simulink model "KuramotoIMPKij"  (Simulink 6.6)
settings: Solver=ode3  StartTime=0.0  StopTime=Tend  FixedStep=dt  RelTol=1e-8
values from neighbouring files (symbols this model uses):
  A0 = [-1/D1 0 0; 0 0 1; 1 0 0]    [PlatoonDemo.m]    (also in SelfOrgCopterDemo.m = OverallSystd.A; SyncDemo.m = [0 1; 0 0]; SyncIMPDemo.m = [Ai Bi*kri; SyncKuramotoDemo.m = A01)
  B0 = [1/D1; 0; 0]    [PlatoonDemo.m]    (also in SelfOrgCopterDemo.m = OverallSystd.B; SyncDemo.m = [ke1; kr*br1]; SyncIMPDemo.m = [Bi*kei; 1]; SyncKuramotoDemo.m = B01)
  C0 = 0.00001    (= 1e-05)    [LCNetworkDemo.m]    (also in SyncDemo.m; SyncIMPDemo.m = [Ci 0]; SyncKuramotoDemo.m = C01; SyncMotor.m = [C01 zeros(1,n+1); zeros(1,n+1) C02])
  D0 = 0    [SyncDemo.m]    (also in SyncIMPDemo.m; SyncKuramotoDemo.m; SyncMotor.m)
  K = [0:kend-1]    [ConvergenceDemo.m]    (also in DelayDemo.m = inv(diag(-diag(K)))*K; EventtriggeredPendulum.m = lqr(invPendel,q*Q, R, 0); SelfOrgCopterDemo.m = Kneighb; SyncDemo.m = [1 1])
  k = k+1    (= 1)    [charPathLength.m]    (also in SyncKuramotoDemo.m = 0.2)
  n = na+1    (= 3)    [DelayDemo.m]    (also in EventtriggeredPendulum.m = 4; LCLCNetworkDemo.m = 4; LCNetworkDemo.m = 2; PlatoonDemo.m)
  Ni = sum(K')    [SyncKuramotoDemo.m]
  x0 = x0/sum(x0)*N1    [ConsensusDemo.m]    (also in EventtriggeredPendulum.m = [0; 0.18; 0; 0]; LCLCNetworkDemo.m = [x01; zeros((N1-1)*n, 1)]; LCNetworkDemo.m = [1 0 0.5 0 -1 0]; NetwPendulum.m = [0; 0; 0.05; 0])

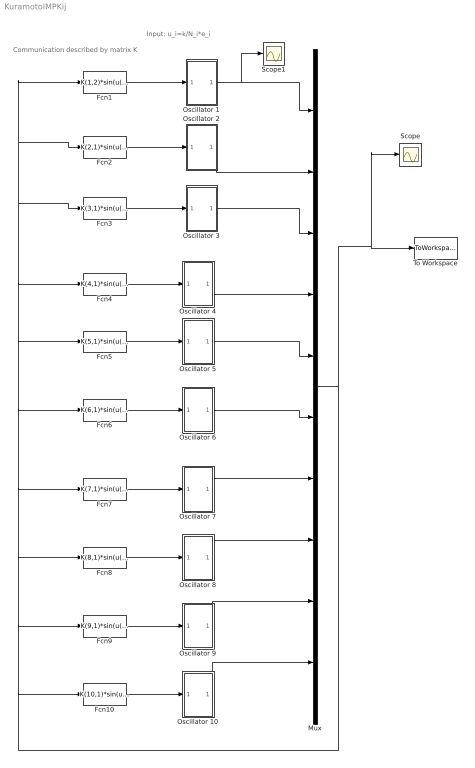
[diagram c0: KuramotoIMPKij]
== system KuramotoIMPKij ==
  note: Communication described by matrix K
  note: Input: u_i=k/N_i*e_i
  Fcn1 : Fcn  Expr=K(1,2)*sin(u(2)-u(1))+K(1,3)*sin(u(3)-u(1))+K(1,4)*sin(u(4)-u(1))+K(1,5)*sin(u(5)-u(1))+K(1,6)*sin(u(6)-u(1))+K(1,7)*sin(u(7)-u(1))+K(1,8)*sin(u(8)-u(1))+K(1,9)*sin(u(9)-u(1))+K(1,10)*sin(u(10)-u(1))
  Fcn10 : Fcn  Expr=K(10,1)*sin(u(1)-u(10))+K(10,2)*sin(u(2)-u(10))+K(10,3)*sin(u(3)-u(10))+K(10,4)*sin(u(4)-u(10))+K(10,5)*sin(u(5)-u(10))+K(10,6)*sin(u(6)-u(10))+K(10,7)*sin(u(7)-u(10))+K(10,8)*sin(u(8)-u(10))+K(10,9)*sin(u(9)-u(10))
  Fcn2 : Fcn  Expr=K(2,1)*sin(u(1)-u(2))+K(2,3)*sin(u(3)-u(2))+K(2,4)*sin(u(4)-u(2))+K(2,5)*sin(u(5)-u(2))+K(2,6)*sin(u(6)-u(2))+K(2,7)*sin(u(7)-u(2))+K(2,8)*sin(u(8)-u(2))+K(2,9)*sin(u(9)-u(2))+K(2,10)*sin(u(10)-u(2))
  Fcn3 : Fcn  Expr=K(3,1)*sin(u(1)-u(3))+K(3,2)*sin(u(2)-u(3))+K(3,4)*sin(u(4)-u(3))+K(3,5)*sin(u(5)-u(3))+K(3,6)*sin(u(6)-u(3))+K(3,7)*sin(u(7)-u(3))+K(3,8)*sin(u(8)-u(3))+K(3,9)*sin(u(9)-u(3))+K(3,10)*sin(u(10)-u(3))
  Fcn4 : Fcn  Expr=K(4,1)*sin(u(1)-u(4))+K(4,2)*sin(u(2)-u(4))+K(4,3)*sin(u(3)-u(4))+K(4,5)*sin(u(5)-u(4))+K(4,6)*sin(u(6)-u(4))+K(4,7)*sin(u(7)-u(4))+K(4,8)*sin(u(8)-u(4))+K(4,9)*sin(u(9)-u(4))+K(4,10)*sin(u(10)-u(4))
  Fcn5 : Fcn  Expr=K(5,1)*sin(u(1)-u(5))+K(5,2)*sin(u(2)-u(5))+K(5,3)*sin(u(3)-u(5))+K(5,4)*sin(u(4)-u(5))+K(5,6)*sin(u(6)-u(5))+K(5,7)*sin(u(7)-u(5))+K(5,8)*sin(u(8)-u(5))+K(5,9)*sin(u(9)-u(5))+K(5,10)*sin(u(10)-u(5))
  Fcn6 : Fcn  Expr=K(6,1)*sin(u(1)-u(6))+K(6,2)*sin(u(2)-u(6))+K(6,3)*sin(u(3)-u(6))+K(6,4)*sin(u(4)-u(6))+K(6,5)*sin(u(5)-u(6))+K(6,7)*sin(u(7)-u(6))+K(6,8)*sin(u(8)-u(6))+K(6,9)*sin(u(9)-u(6))+K(6,10)*sin(u(10)-u(6))
  Fcn7 : Fcn  Expr=K(7,1)*sin(u(1)-u(7))+K(7,2)*sin(u(2)-u(7))+K(7,3)*sin(u(3)-u(7))+K(7,4)*sin(u(4)-u(7))+K(7,5)*sin(u(5)-u(7))+K(7,6)*sin(u(6)-u(7))+K(7,8)*sin(u(8)-u(7))+K(7,9)*sin(u(9)-u(7))+K(7,10)*sin(u(10)-u(7))
  Fcn8 : Fcn  Expr=K(8,1)*sin(u(1)-u(8))+K(8,2)*sin(u(2)-u(8))+K(8,3)*sin(u(3)-u(8))+K(8,4)*sin(u(4)-u(8))+K(8,5)*sin(u(5)-u(8))+K(8,6)*sin(u(6)-u(8))+K(8,7)*sin(u(7)-u(8))+K(8,9)*sin(u(9)-u(8))+K(8,10)*sin(u(10)-u(8))
  Fcn9 : Fcn  Expr=K(9,1)*sin(u(1)-u(9))+K(9,2)*sin(u(2)-u(9))+K(9,3)*sin(u(3)-u(9))+K(9,4)*sin(u(4)-u(9))+K(9,5)*sin(u(5)-u(9))+K(9,6)*sin(u(6)-u(9))+K(9,7)*sin(u(7)-u(9))+K(9,8)*sin(u(8)-u(9))+K(9,10)*sin(u(10)-u(9))
  Mux : Mux  Inputs=10
  Oscillator 1 : Subsystem
  Oscillator 10 : Subsystem
  Oscillator 2 : Subsystem
  Oscillator 3 : Subsystem
  Oscillator 4 : Subsystem
  Oscillator 5 : Subsystem
  Oscillator 6 : Subsystem
  Oscillator 7 : Subsystem
  Oscillator 8 : Subsystem
  Oscillator 9 : Subsystem
  Scope : Scope
  Scope1 : Scope
  To Workspace : ToWorkspace  VariableName=Theta  SampleTime=-1  SaveFormat=Array
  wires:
  Oscillator 1/1(y_1) -> Mux/1, Scope1/1
  Oscillator 2/1(y_2) -> Mux/2
  Oscillator 3/1(y_3) -> Mux/3
  Oscillator 4/1(y_4) -> Mux/4
  Oscillator 5/1(y_5) -> Mux/5
  Oscillator 6/1(y_6) -> Mux/6
  Mux/1 -> To Workspace/1, Scope/1, Fcn1/1, Fcn2/1, Fcn3/1, Fcn4/1, Fcn5/1, Fcn6/1, Fcn7/1, Fcn8/1, Fcn9/1, Fcn10/1
  Fcn1/1 -> Oscillator 1/1(e_1)
  Fcn2/1 -> Oscillator 2/1(e_2)
  Fcn3/1 -> Oscillator 3/1(e_3)
  Fcn4/1 -> Oscillator 4/1(e_4)
  Fcn5/1 -> Oscillator 5/1(e_5)
  Fcn6/1 -> Oscillator 6/1(e_6)
  Oscillator 7/1(y_7) -> Mux/7
  Oscillator 8/1(y_8) -> Mux/8
  Oscillator 9/1(y_9) -> Mux/9
  Oscillator 10/1(y_10) -> Mux/10
  Fcn10/1 -> Oscillator 10/1(e_10)
  Fcn9/1 -> Oscillator 9/1(e_9)
  Fcn8/1 -> Oscillator 8/1(e_8)
  Fcn7/1 -> Oscillator 7/1(e_7)

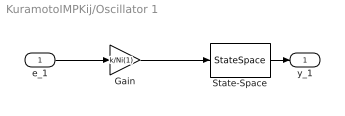
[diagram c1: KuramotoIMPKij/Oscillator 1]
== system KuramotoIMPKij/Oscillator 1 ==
  e_1 : Inport
  Gain : Gain  Gain=k/Ni(1)
  State-Space : StateSpace  A=A0  B=B0  C=C0  D=D0  X0=x0(1:n)
  y_1 : Outport
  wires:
  e_1/1 -> Gain/1
  State-Space/1 -> y_1/1
  Gain/1 -> State-Space/1

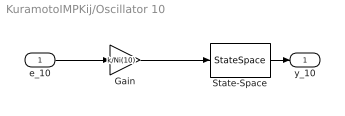
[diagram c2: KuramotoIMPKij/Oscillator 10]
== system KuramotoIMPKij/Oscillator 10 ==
  e_10 : Inport
  Gain : Gain  Gain=k/Ni(10)
  State-Space : StateSpace  A=A0  B=B0  C=C0  D=D0  X0=x0(9*n+1:10*n)
  y_10 : Outport
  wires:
  e_10/1 -> Gain/1
  State-Space/1 -> y_10/1
  Gain/1 -> State-Space/1

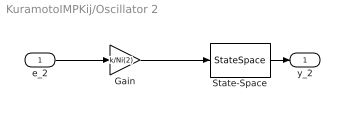
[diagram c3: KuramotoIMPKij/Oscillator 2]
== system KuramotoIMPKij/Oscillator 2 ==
  e_2 : Inport
  Gain : Gain  Gain=k/Ni(2)
  State-Space : StateSpace  A=A0  B=B0  C=C0  D=D0  X0=x0(n+1:2*n)
  y_2 : Outport
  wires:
  e_2/1 -> Gain/1
  State-Space/1 -> y_2/1
  Gain/1 -> State-Space/1

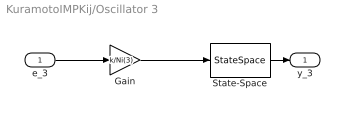
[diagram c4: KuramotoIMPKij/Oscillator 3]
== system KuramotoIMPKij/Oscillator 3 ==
  e_3 : Inport
  Gain : Gain  Gain=k/Ni(3)
  State-Space : StateSpace  A=A0  B=B0  C=C0  D=D0  X0=x0(2*n+1:3*n)
  y_3 : Outport
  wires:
  e_3/1 -> Gain/1
  State-Space/1 -> y_3/1
  Gain/1 -> State-Space/1

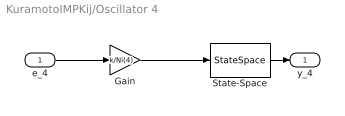
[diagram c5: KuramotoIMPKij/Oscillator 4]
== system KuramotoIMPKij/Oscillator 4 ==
  e_4 : Inport
  Gain : Gain  Gain=k/Ni(4)
  State-Space : StateSpace  A=A0  B=B0  C=C0  D=D0  X0=x0(3*n+1:4*n)
  y_4 : Outport
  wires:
  e_4/1 -> Gain/1
  State-Space/1 -> y_4/1
  Gain/1 -> State-Space/1

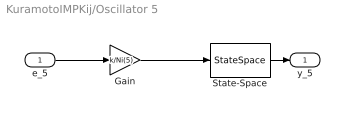
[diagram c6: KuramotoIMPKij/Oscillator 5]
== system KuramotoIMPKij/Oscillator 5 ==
  e_5 : Inport
  Gain : Gain  Gain=k/Ni(5)
  State-Space : StateSpace  A=A0  B=B0  C=C0  D=D0  X0=x0(4*n+1:5*n)
  y_5 : Outport
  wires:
  e_5/1 -> Gain/1
  State-Space/1 -> y_5/1
  Gain/1 -> State-Space/1

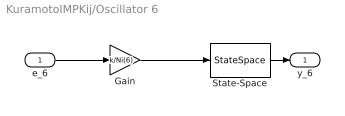
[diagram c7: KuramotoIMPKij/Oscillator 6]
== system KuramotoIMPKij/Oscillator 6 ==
  e_6 : Inport
  Gain : Gain  Gain=k/Ni(6)
  State-Space : StateSpace  A=A0  B=B0  C=C0  D=D0  X0=x0(5*n+1:6*n)
  y_6 : Outport
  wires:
  e_6/1 -> Gain/1
  State-Space/1 -> y_6/1
  Gain/1 -> State-Space/1

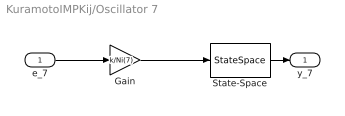
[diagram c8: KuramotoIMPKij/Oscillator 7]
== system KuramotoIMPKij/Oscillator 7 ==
  e_7 : Inport
  Gain : Gain  Gain=k/Ni(7)
  State-Space : StateSpace  A=A0  B=B0  C=C0  D=D0  X0=x0(6*n+1:7*n)
  y_7 : Outport
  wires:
  e_7/1 -> Gain/1
  State-Space/1 -> y_7/1
  Gain/1 -> State-Space/1

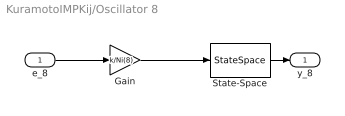
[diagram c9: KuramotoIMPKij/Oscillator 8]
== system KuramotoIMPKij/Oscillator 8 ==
  e_8 : Inport
  Gain : Gain  Gain=k/Ni(8)
  State-Space : StateSpace  A=A0  B=B0  C=C0  D=D0  X0=x0(7*n+1:8*n)
  y_8 : Outport
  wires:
  e_8/1 -> Gain/1
  State-Space/1 -> y_8/1
  Gain/1 -> State-Space/1

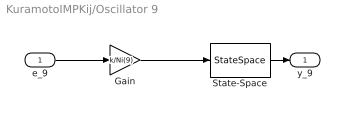
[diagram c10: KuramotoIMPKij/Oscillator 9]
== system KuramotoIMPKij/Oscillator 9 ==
  e_9 : Inport
  Gain : Gain  Gain=k/Ni(9)
  State-Space : StateSpace  A=A0  B=B0  C=C0  D=D0  X0=x0(8*n+1:9*n)
  y_9 : Outport
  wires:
  e_9/1 -> Gain/1
  State-Space/1 -> y_9/1
  Gain/1 -> State-Space/1
